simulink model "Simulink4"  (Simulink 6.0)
settings: Solver=ode45  StartTime=0.0  StopTime=60  RelTol=1e-3
libraries: simulink_extras x1

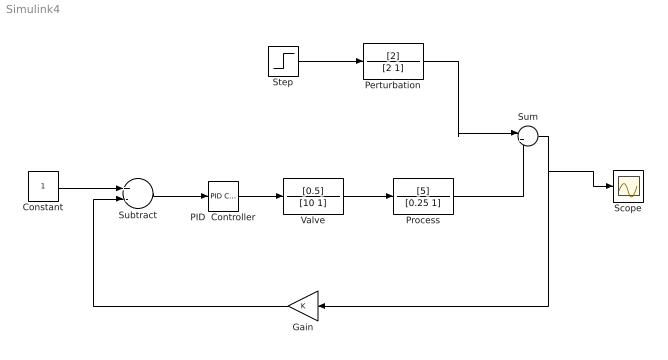
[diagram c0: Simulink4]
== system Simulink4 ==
  Constant : Constant
  Gain : Gain  Orientation=left
  PID  Controller : simulink_extras/Additional Linear/PID Controller  P=1  I=1  D=0
  Perturbation : TransferFcn  Numerator=[2]  Denominator=[2 1]
  Process : TransferFcn  Numerator=[5]  Denominator=[0.25 1]
  Scope : Scope
  Step : Step  SampleTime=0
  Subtract : Sum  Inputs=+-  OutScaling=2^-10
  Sum : Sum  Inputs=|++
  Valve : TransferFcn  Numerator=[0.5]  Denominator=[10 1]
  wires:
  Constant/1 -> Subtract/1
  Subtract/1 -> PID  Controller/1
  PID  Controller/1 -> Valve/1
  Valve/1 -> Process/1
  Process/1 -> Sum/2
  Step/1 -> Perturbation/1
  Perturbation/1 -> Sum/1
  Sum/1 -> Gain/1, Scope/1
  Gain/1 -> Subtract/2
